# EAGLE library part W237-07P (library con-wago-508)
WAGO SREW CLAMP
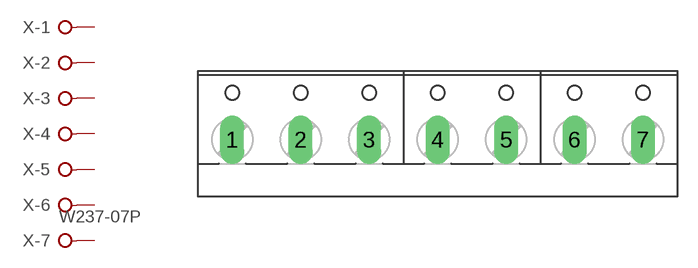
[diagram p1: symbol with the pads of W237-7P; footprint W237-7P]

Designator prefix X; gates -1=KL -2=KL -3=KL -4=KL -5=KL -6=KL -7=KL+V

## W237-07P (OC_FARNELL: unknown; OC_NEWARK: unknown)  [W237-7P]
1  -1:KL  pas
2  -2:KL  pas
3  -3:KL  pas
4  -4:KL  pas
5  -5:KL  pas
6  -6:KL  pas
7  -7:KL  pas

## Footprint W237-7P (pad centres in mm)
WAGO SREW CLAMP
drill 1.194 long: 1 -15.24,-0.635; 2 -10.16,-0.635; 3 -5.08,-0.635; 4 0,-0.635; 5 5.08,-0.635; 6 10.16,-0.635; 7 15.24,-0.635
